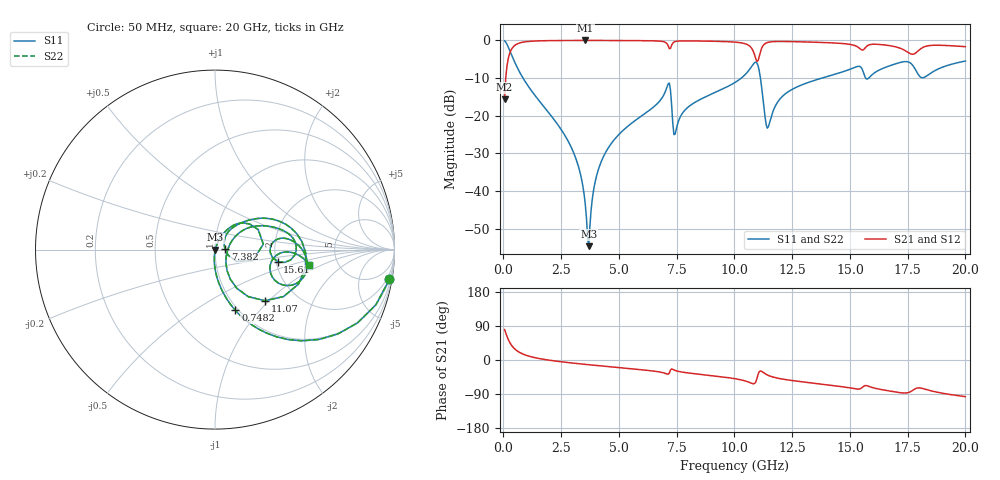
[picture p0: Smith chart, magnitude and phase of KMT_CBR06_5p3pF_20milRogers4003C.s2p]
! Data measured by Modelithics Inc. support@modelithics.com 813-866-6335
! KEMET CBR0603 5.3pF, Pad Width= 0.851mm, Pad Length= 0.64mm, Pad Gap= 0.62mm, 20mil Rogers 4003C substrate Data, January 2022
# hz S ma R 50
! 2 Port Network Data from SP1.SP block
! freq  magS11  angS11  magS21  angS21  magS12  angS12  magS22  angS22
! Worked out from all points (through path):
!   401 points, 50 MHz to 20 GHz, reference 50 ohm
!   highest |S21| = -0.02 dB at 3.541 GHz (marker M1); lowest = -15.6 dB at 50 MHz (marker M2)
!   group delay of S21, straight-line fit = 15.3 ps
!   lowest |S11| = -54.6 dB at 3.691 GHz (marker M3), VSWR 1.00, Z = 50.2 + j0.0126 ohm
!   |S11| at or under -10 dB: 847.6 MHz to 10.3 GHz (9.449 GHz wide, 170 % of centre); 11.13 GHz to 13.79 GHz (2.661 GHz wide, 21.4 % of centre); 15.69 GHz to 15.81 GHz (129.1 MHz wide, 0.82 % of centre)
!   |S22| runs from -54.6 to -0.1 dB; largest |S21 - S12| = 0
!   S11 on the Smith chart (normalised r, x): 50 MHz: 1, -12; 748.2 MHz: 0.97, -0.75; 7.382 GHz: 1.12, +0.00; 11.07 GHz: 1.40, -0.94; 15.61 GHz: 2.04, -0.31; 20 GHz: 3.09, -0.72
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5e7  0.9861 -9.7  0.1656 80.3  0.1656 80.3  0.9861 -9.7
2.99375e8  0.7027 -46.3  0.7108 43.6  0.7108 43.6  0.7027 -46.3
7.4825e8  0.3569 -71.5  0.9332 18.4  0.9332 18.4  0.3569 -71.5
2.74325e9  0.0496 -94.6  0.9971 -6.4  0.9971 -6.4  0.0496 -94.6
3.391625e9  0.01393 -93.6  0.9981 -10.6  0.9981 -10.6  0.01393 -93.6
3.54125e9  0.006757 -86.6  0.9981 -11.5  0.9981 -11.5  0.006757 -86.6
3.690875e9  0.001861 3.9  0.9981 -12.4  0.9981 -12.4  0.001861 3.9
3.990125e9  0.01415 68.2  0.9979 -14.2  0.9979 -14.2  0.01415 68.2
4.439e9  0.0333 69.7  0.9973 -16.8  0.9973 -16.8  0.0333 69.7
6.73325e9  0.1529 55.4  0.9794 -31.3  0.9794 -31.3  0.1529 55.4
7.13225e9  0.2653 24.8  0.8484 -37.4  0.8484 -37.4  0.2653 24.8
7.381625e9  0.05618 1.3  0.9495 -26.2  0.9495 -26.2  0.05618 1.3
1.0025e10  0.2765 38.1  0.9483 -49.3  0.9483 -49.3  0.2765 38.1
1.067338e10  0.419 19.6  0.8334 -59.7  0.8334 -59.7  0.419 19.6
1.107238e10  0.3977 -45.7  0.61 -30.8  0.61 -30.8  0.3977 -45.7
1.147138e10  0.07162 1.6  0.9455 -40.7  0.9455 -40.7  0.07162 1.6
1.206988e10  0.1799 34.7  0.9676 -50.2  0.9676 -50.2  0.1799 34.7
1.336662e10  0.2882 27.5  0.9485 -60.8  0.9485 -60.8  0.2882 27.5
1.5611e10  0.3554 -10.8  0.7638 -68.6  0.7638 -68.6  0.3554 -10.8
1.670825e10  0.4588 3.8  0.8529 -81.7  0.8529 -81.7  0.4588 3.8
1.775562e10  0.4509 -26.4  0.6573 -78.6  0.6573 -78.6  0.4509 -26.4
2e10  0.5323 -9.0  0.8255 -96.8  0.8255 -96.8  0.5323 -9.0
